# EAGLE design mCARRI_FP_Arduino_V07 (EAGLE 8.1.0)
CNAME: RDUINO V4; CREVISION: 4; DESIGNER: RODNEYD

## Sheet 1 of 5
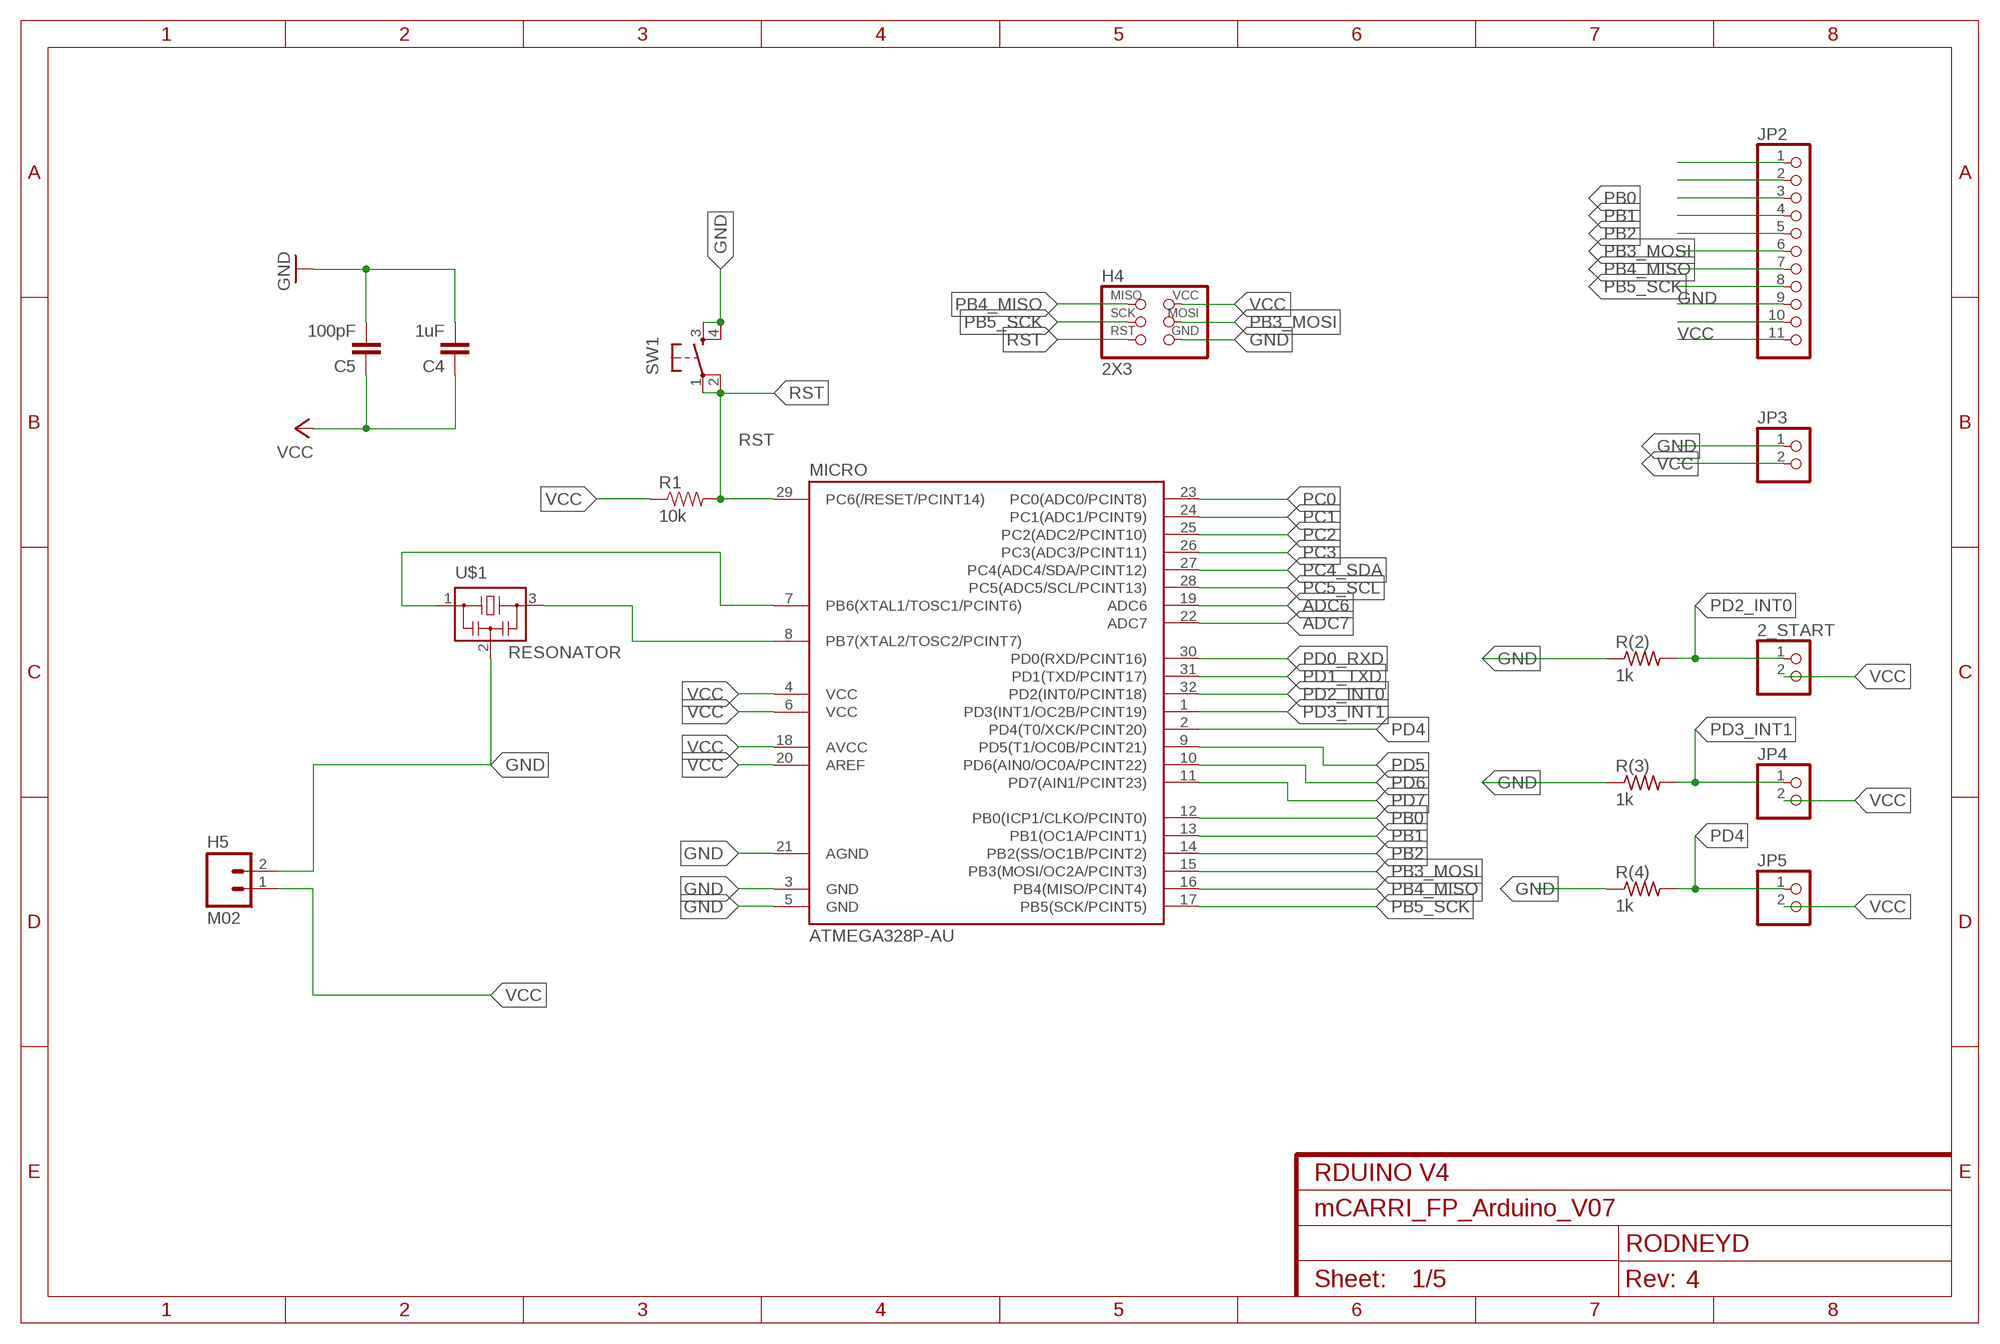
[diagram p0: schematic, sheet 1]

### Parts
2_START  PINHD-1X2  [1X02]
C4  1uF  CAP1206  [1206]
C5  100pF  CAP1206  [1206]
H4  2X3  AVRISPSMD  [2X03SMD]
H5  M02  [1X02_SMD_FLAT_PADS]
JP2  PINHD-1X11  [1X11]
JP3  PINHD-1X2  [1X02]
JP4  PINHD-1X2  [1X02]
JP5  PINHD-1X2  [1X02]
MICRO  ATMEGA328P-AU  ATMEGA48/88/168-AU  [TQFP32-08]
R1  10k  RESISTOR1206  [1206]
R(2)  1k  RES-US1206FAB  [R1206FAB]
R(3)  1k  RES-US1206FAB  [R1206FAB]
R(4)  1k  RES-US1206FAB  [R1206FAB]
SW1  6MM_SWITCH6MM_SWITCH  [6MM_SWITCH]
U$1  RESONATOR  [EFOBM]

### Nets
ADC6: MICRO.19(ADC6)
ADC7: MICRO.22(ADC7)
GND: C4.2 C5.2 H4.6(GND) H5.2 JP2.9 JP3.1 MICRO.3(GND) MICRO.5(GND) MICRO.21(AGND) R(2).1 R(3).1 R(4).1 SW1.3(S) SW1.4(S1) U$1.2
N$2: MICRO.8(PB7(XTAL2/TOSC2/PCINT7)) U$1.3
N$8: JP2.1
N$9: MICRO.7(PB6(XTAL1/TOSC1/PCINT6)) U$1.1
N$10: JP2.2
N$18: JP2.10
PB0: JP2.3 MICRO.12(PB0(ICP1/CLKO/PCINT0))
PB1: JP2.4 MICRO.13(PB1(OC1A/PCINT1))
PB2: JP2.5 MICRO.14(PB2(SS/OC1B/PCINT2))
PB3_MOSI: H4.4(MOSI) JP2.6 MICRO.15(PB3(MOSI/OC2A/PCINT3))
PB4_MISO: H4.1(MISO) JP2.7 MICRO.16(PB4(MISO/PCINT4))
PB5_SCK: H4.3(SCK) JP2.8 MICRO.17(PB5(SCK/PCINT5))
PC0: MICRO.23(PC0(ADC0/PCINT8))
PC1: MICRO.24(PC1(ADC1/PCINT9))
PC2: MICRO.25(PC2(ADC2/PCINT10))
PC3: MICRO.26(PC3(ADC3/PCINT11))
PC4_SDA: MICRO.27(PC4(ADC4/SDA/PCINT12))
PC5_SCL: MICRO.28(PC5(ADC5/SCL/PCINT13))
PD0_RXD: MICRO.30(PD0(RXD/PCINT16))
PD1_TXD: MICRO.31(PD1(TXD/PCINT17))
PD2_INT0: 2_START.1 MICRO.32(PD2(INT0/PCINT18)) R(2).2
PD3_INT1: JP4.1 MICRO.1(PD3(INT1/OC2B/PCINT19)) R(3).2
PD4: JP5.1 MICRO.2(PD4(T0/XCK/PCINT20)) R(4).2
PD5: MICRO.9(PD5(T1/OC0B/PCINT21))
PD6: MICRO.10(PD6(AIN0/OC0A/PCINT22))
PD7: MICRO.11(PD7(AIN1/PCINT23))
RST: H4.5(RST) MICRO.29(PC6(/RESET/PCINT14)) R1.2 SW1.1(P) SW1.2(P1)
VCC: 2_START.2 C4.1 C5.1 H4.2(VCC) H5.1 JP2.11 JP3.2 JP4.2 JP5.2 MICRO.4(VCC) MICRO.6(VCC) MICRO.18(AVCC) MICRO.20(AREF) R1.1

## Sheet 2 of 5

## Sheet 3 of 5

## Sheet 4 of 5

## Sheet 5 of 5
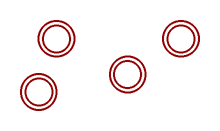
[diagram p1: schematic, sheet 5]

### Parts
U$7  MOUNTINGHOLE2.5  [MOUNTINGHOLE_2.5_PLATED]
U$8  MOUNTINGHOLE2.5  [MOUNTINGHOLE_2.5_PLATED]
U$9  MOUNTINGHOLE2.5  [MOUNTINGHOLE_2.5_PLATED]
U$10  MOUNTINGHOLE2.5  [MOUNTINGHOLE_2.5_PLATED]

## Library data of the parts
2_START JP3-JP5 = pinhead:PINHD-1X2: PIN HEADER
C4 C5 = 01_SparkFun:CAP: Capacitor
H4 = fab:AVRISP
H5 = Working:M02
JP2 = pinhead:PINHD-1X11: PIN HEADER
MICRO = atmega8:ATMEGA48/88/168
R1 = 01_SparkFun:RESISTOR: Resistor
R(2) R(3) R(4) = 01_fab:RES-US: Resistor (US Symbol)
SW1 = 01_FAB_Hello:6MM_SWITCH: OMRON SWITCH
U$1 = fab:RESONATOR
U$7-U$10 = microbuilder:MOUNTINGHOLE: Mounting Hole; BOM: EXCLUDE

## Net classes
1 power: width 0.406 mm

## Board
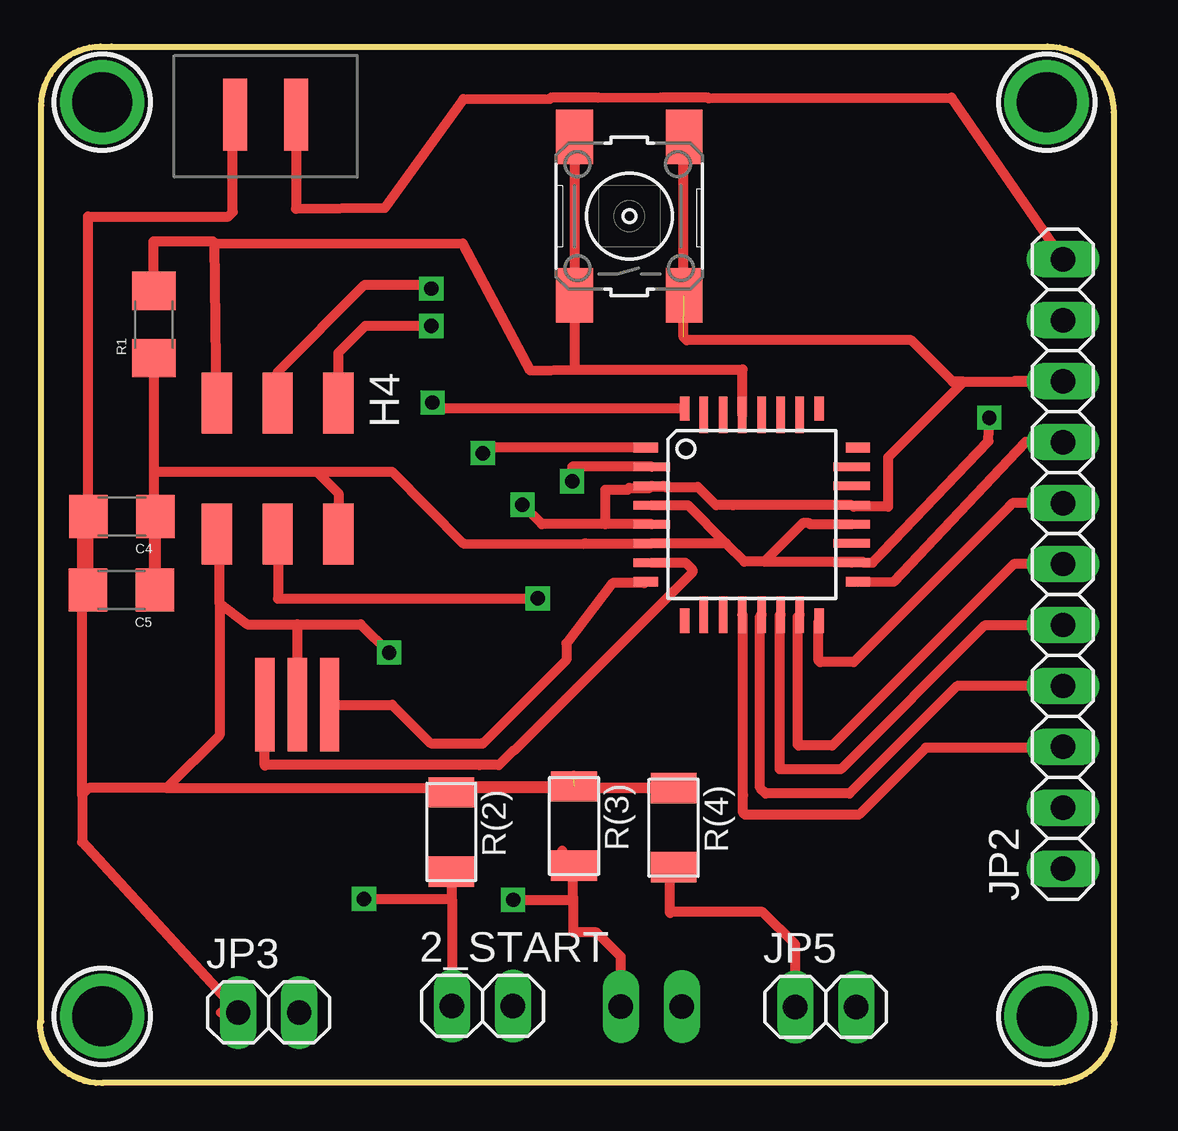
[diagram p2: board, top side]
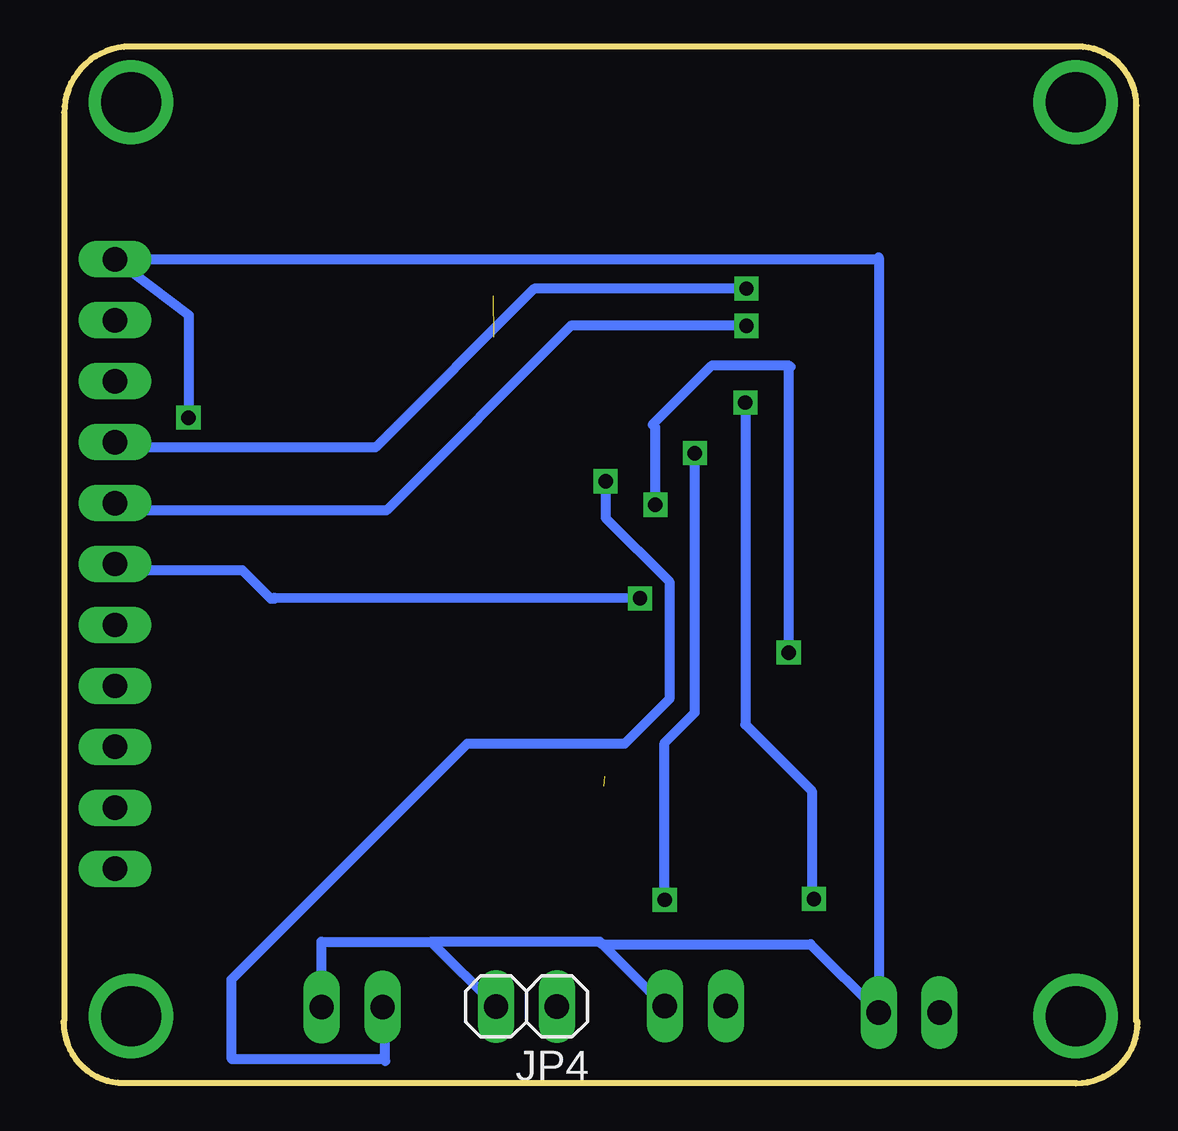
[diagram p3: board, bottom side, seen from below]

No outline drawn. Coordinates in mm, seen from the top.
Copper layers (1*16): Top 0.035mm / dielectric 1.5mm / Bottom 0.035mm
Design rules "default *": minimum track width 12mil, minimum drill 24mil, track to track 12mil, track to pad 12mil, pad to pad 8mil, via to via 8mil, smd to smd 8mil, copper to edge 40mil, drill to drill 2mil, minimum pad ring 10mil, minimum via ring 8mil, stop-mask expansion 4mil, vias tented up to drill 0mil, thermal gap 10mil
Milling: 14 lines

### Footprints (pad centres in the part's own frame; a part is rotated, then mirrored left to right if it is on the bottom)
1X02 = drill 1.016 long: 1 -1.27,0; 2 1.27,0
1206 = smd 1.6 x 1.8: 1 -1.4,0; 2 1.4,0
2X03SMD = smd 2.54 x 1.27: 1 -2.54,2.54; 2 2.92,2.54; 3 -2.54,0; 4 2.92,0; 5 -2.54,-2.54; 6 2.92,-2.54
1X02_SMD_FLAT_PADS = smd 1 x 3: 1 2.54,1.19; 2 5.08,1.19
1X11 = drill 1.016 long: 1 -12.7,0; 2 -10.16,0; 3 -7.62,0; 4 -5.08,0; 5 -2.54,0; 6 0,0; 7 2.54,0; 8 5.08,0; 9 7.62,0; 10 10.16,0; 11 12.7,0
TQFP32-08 = smd 1.016 x 0.406: 1 -4.42,2.8; 8 -4.42,-2.8; 17 4.42,-2.8; 24 4.42,2.8 | smd 1.524 x 0.356: 2 -4.166,2; 3 -4.166,1.2; 4 -4.166,0.4; 5 -4.166,-0.4; 6 -4.166,-1.2; 7 -4.166,-2; 18 4.166,-2; 19 4.166,-1.2; 20 4.166,-0.4; 21 4.166,0.4; 22 4.166,1.2; 23 4.166,2 | smd 0.406 x 1.016: 9 -2.8,-4.42; 16 2.8,-4.42; 25 2.8,4.42; 32 -2.8,4.42 | smd 0.356 x 1.524: 10 -2,-4.166; 11 -1.2,-4.166; 12 -0.4,-4.166; 13 0.4,-4.166; 14 1.2,-4.166; 15 2,-4.166; 26 2,4.166; 27 1.2,4.166; 28 0.4,4.166; 29 -0.4,4.166; 30 -1.2,4.166; 31 -2,4.166
R1206FAB = smd 1.27 x 1.905: 1 -1.651,0; 2 1.651,0
6MM_SWITCH = smd 2.286 x 1.524: 1 -3.302,2.286; 2 3.302,2.286; 3 -3.302,-2.286; 4 3.302,-2.286
EFOBM = smd 0.8 x 3.9: 1 -1.35,0; 2 0,0; 3 1.35,0
MOUNTINGHOLE_2.5_PLATED = drill 2.5 pad 3.2: P$1 0,0

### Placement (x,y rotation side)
2_START  18.86,3.45 0 top
C4  3.83,23.86 180 top
C5  3.82,20.79 180 top
H4  10.32,26.05 270 top
H5  13.64,41.8 180 top
JP2  43.06,21.87 90 top
JP3  9.95,3.18 0 top
JP4  25.9,3.43 180 bottom
JP5  33.17,3.41 0 top
MICRO  30.09,23.93 0 top
R1  5.17,31.85 90 top
R(2)  17.56,10.7 270 top
R(3)  22.68,10.95 270 top
R(4)  26.83,10.88 270 top
SW1  24.99,36.37 90 top
U$1  11.15,16 0 top
U$7  3.01,41.12 0 top
U$8  3.01,3.02 0 top
U$9  42.38,41.12 0 top
U$10  42.38,3.02 0 top

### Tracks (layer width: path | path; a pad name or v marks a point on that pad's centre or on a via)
GND  (via drill 0.6)  (2 unrouted)
  Top 0.406: H5.2 8.6,40.57 | H5.2 8.63,40.61 | 41.02,29.49 JP2.9 43.04,29.47 38.93,29.47 | 26.45,25.08 27.84,25.08 28.6,24.32 29.3,24.32 29.31,24.33 MICRO.21 34.33,24.26 35.78,24.26 35.78,26.32 38.93,29.47 | 26.45,25.08 25.98,25.08 MICRO.3 25.84,25.04 24.98,25.04 24.91,24.97 23.98,24.97 23.98,23.53 | 26.4,25.13 26.45,25.08 | 7.96,3.18 JP3.1 | 38.93,29.47 38.47,29.47 36.74,31.2 27.37,31.2 27.25,31.32 27.25,39.65 SW1.4 | 7.9,20.23 9.06,19.36 11.15,19.36 | 7.9,20.23 7.9,23.01 H4.6 | JP3.1 | JP3.1 2.17,10.28 | 2.17,10.27 2.17,10.28 | 2.17,12.26 2.17,12.67 | 2.17,12.26 2.17,10.28 | 2.17,12.67 2.17,13.01 2.17,23.71 C4.2 | 11.34,16 U$1.2 11.15,19.36 | MICRO.5 23.98,23.53 | 22.67,13.04 22.64,13.01 | 2.2,12.64 2.17,12.67 | C4.2 2.44,36.34 2.42,36.36 8.27,36.36 8.45,36.54 8.45,40.5 H5.2 | C4.2 2.44,20.8 C5.2 | 5.7,12.53 R(4).1 22.75,12.53 R(3).1 17.81,12.6 R(2).1 | 5.7,12.53 2.44,12.53 2.17,12.26 | 7.9,20.23 7.9,14.73 5.7,12.53 | 23.98,23.53 21.34,23.53 v20.53,24.34 | 11.15,19.36 13.79,19.36 v14.97,18.18
  Bottom 0.406: v20.53,24.34 20.53,27.57 20.64,27.68 18.18,30.14 14.94,30.14 | 14.94,30.14 14.89,30.09 | v14.97,18.18 14.97,30.11 14.94,30.14
N$2
  Top 0.406: MICRO.8 25.61,21.07 24.29,21.07 22.36,18.56 22.36,17.88 18.86,14.38 18.84,14.4 16.71,14.4 15.11,16 U$1.3 12.54,16.05
N$9
  Top 0.406: MICRO.7 27.32,21.93 27.61,21.64 27.61,21.52 20.17,14.08 20.14,14.08 19.55,13.49 18.73,13.49 18.72,13.49 9.81,13.49 9.79,13.47 U$1.1
PB0
  Top 0.406: JP2.3 43.02,14.21 37.34,14.21 34.55,11.42 29.81,11.42 29.73,11.5 29.73,12.23 29.72,12.24 29.72,19.74 MICRO.12
PB1
  Top 0.406: JP2.4 38.64,16.78 34.16,12.3 30.67,12.3 30.43,12.54 30.43,19.7 MICRO.13
PB2
  Top 0.406: JP2.5 43.03,19.3 39.79,19.3 33.8,13.31 31.26,13.31 31.26,19.73 MICRO.14
PB3_MOSI  (via drill 0.6)
  Top 0.406: JP2.6 41.01,21.87 33.44,14.3 32.05,14.3 32,14.35 32,19.68 MICRO.15 | H4.4 10.34,23.12 10.34,20.43 20.8,20.43 v21.17,20.44
  Bottom 0.406: v21.17,20.44 36.41,20.46 36.41,20.42 36.55,20.42 37.74,21.61 42.8,21.61 JP2.6
PB4_MISO  (via drill 0.6)
  Top 0.406: JP2.7 40.95,24.41 40.84,24.3 40.84,24.28 34.34,17.78 32.94,17.78 32.87,17.85 32.87,19.49 MICRO.16 | H4.1 12.87,30.68 13.99,31.8 v16.73,31.8
  Bottom 0.406: v16.73,31.8 24.05,31.8 31.74,24.11 42.76,24.11 JP2.7
PB5_SCK  (via drill 0.6)
  Top 0.406: MICRO.17 36.01,21.14 41.5,26.96 JP2.8 | H4.3 10.32,29.88 13.96,33.51 16.57,33.51 v16.73,33.35
  Bottom 0.406: v16.73,33.35 25.58,33.35 32.2,26.73 42.84,26.73 JP2.8
PD2_INT0  (via drill 0.6)
  Top 0.406: 17.53,3.51 2_START.1 17.59,7.89 | 17.59,7.89 17.59,8.98 R(2).2 | MICRO.32 17.03,28.35 v16.78,28.6 | v13.92,7.91 17.57,7.91 17.59,7.89
  Bottom 0.406: v16.78,28.6 16.78,15.18 14.01,12.41 14.01,8 v13.92,7.91
PD3_INT1  (via drill 0.6)
  Top 0.406: 24.81,3.61 JP4.1 24.63,5.5 23.62,6.51 22.66,6.51 22.64,6.53 22.64,7.97 | 22.64,7.97 22.64,8.91 R(3).2 22.19,9.92 | MICRO.1 19.12,26.73 v18.88,26.49 | v20.14,7.87 22.54,7.87 22.64,7.97
  Bottom 0.406: v18.88,26.49 18.88,15.68 18.9,15.66 20.14,14.42 v20.14,7.87
PD4  (via drill 0.6)
  Top 0.406: 32.05,3.56 JP5.1 31.9,6.01 30.54,7.37 26.74,7.37 26.68,7.31 26.68,8.86 R(4).2 | MICRO.2 22.6,25.93 v22.6,25.32
  Bottom 0.406: v22.6,25.32 22.6,23.79 19.95,21.14 19.95,16.24 21.81,14.38 28.37,14.38 38.21,4.54 38.21,1.28 38.17,1.24 31.87,1.24 31.79,1.16 31.79,3.3 JP5.1
RST
  Top 0.406: MICRO.29 29.7,29.98 22.71,29.98 | 22.71,29.98 SW1.1 SW1.2 | 7.71,35.24 18.04,35.23 20.85,29.94 22.71,29.98 | H4.5 7.71,35.24 | R1.2 5.17,35.3 5.14,35.32 7.63,35.32 7.71,35.24
VCC  (via drill 0.6)
  Top 0.406: 11.06,40.61 H5.1 11.09,36.68 14.8,36.72 18.07,41.25 21.66,41.26 21.73,41.32 23.67,41.32 23.68,41.31 26.3,41.32 28.24,41.32 28.29,41.28 38.41,41.31 JP2.11 | 34.76,21.93 MICRO.18 | 34.76,21.93 35.12,21.93 35.53,22.34 35.53,22.37 39.96,26.99 v39.99,27.97 39.86,27.79 | MICRO.4 27.42,24.33 29.02,22.73 | 29.02,22.73 29.78,21.97 30.62,21.97 | 30.62,21.97 34.72,21.97 34.76,21.93 | MICRO.20 32.52,23.53 32.48,23.57 32.22,23.57 30.62,21.97 | 29.02,22.73 MICRO.6 23.14,22.73 23.08,22.71 18.06,22.73 15.09,25.72 11.96,25.72 | H4.2 12.87,24.81 11.96,25.72 | R1.1 5.17,25.72 | 5.17,25.72 5.17,20.84 C5.1 5.24,20.8 C4.1 | 5.17,25.72 11.96,25.72
  Bottom 0.406: v39.99,27.97 39.98,32.24 JP2.11 11.3,34.57 11.22,34.65 JP3.2 14.06,6.02 22.74,6.02 | JP5.2 34.44,6.13 29.87,6.13 | 29.87,6.13 JP4.2 | 29.87,6.13 22.85,6.13 22.74,6.02 | 2_START.2 20.17,3.45 22.74,6.02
